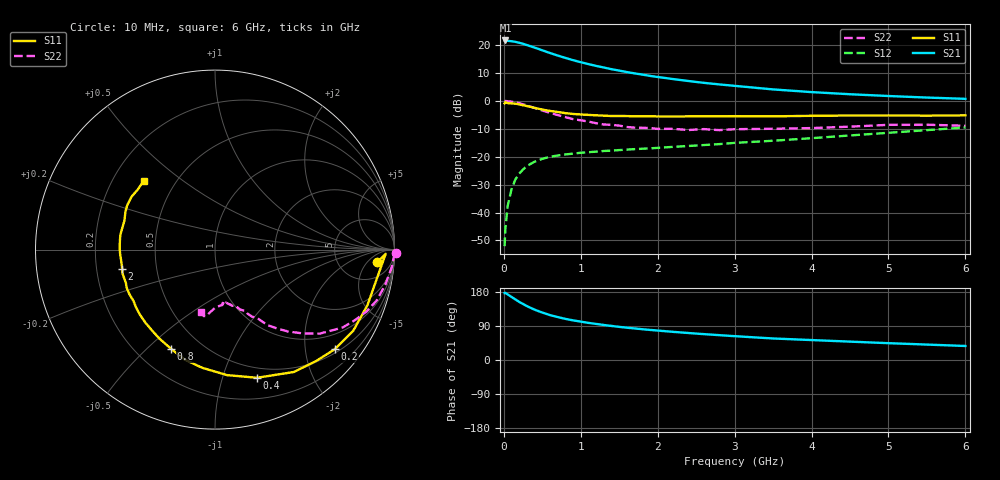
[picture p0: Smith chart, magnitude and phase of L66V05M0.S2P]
!  INFINEON TECHNOLOGIES Small Signal Semiconductors
! BFR380L3 , Si-NPN RF-Transistor in TSLP-3-1
!  Vce=6 V,  Ic=5 mA
! Common Emitter S-Parameters:  07. March 2005
#  GHz  S  MA  R  50
! f  S11  S21  S12  S22
! GHz  Mag  Ang  Mag  Ang  Mag  Ang  Mag  Ang
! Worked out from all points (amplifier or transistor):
!   36 points, 10 MHz to 6 GHz, reference 50 ohm
!   highest |S21| = 21.7 dB at 20 MHz (marker M1)
!   |S21| within 3 dB of that: start of sweep to 445.7 MHz
!   unconditionally stable (mu >= 1): 3.068 GHz to 4.502 GHz
!   at 250 MHz: K = 0.14, MSG = 22.5 dB, |S12| = -24.6 dB
!   at 1.4 GHz: K = 0.69, MSG = 14.6 dB, |S12| = -17.8 dB
!   at 6 GHz: K = 0.92, MSG = 5.1 dB, |S12| = -9.5 dB
!   S11 on the Smith chart (normalised r, x): 10 MHz: 13, -10; 200 MHz: 0.59, -2.65; 400 MHz: 0.40, -1.30; 800 MHz: 0.34, -0.60; 2 GHz: 0.31, -0.09; 6 GHz: 0.33, +0.37
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0.01  0.9068 -4.4  12.08 176.7  0.0025 71.3  1.011 -1.2
0.02  0.9514 -1.4  12.13 177.3  0.0051 91.3  0.997 -2.5
0.05  0.9152 -10.5  11.97 173.0  0.0132 85.6  0.9886 -6.0
0.1  0.9042 -20.0  11.73 166.4  0.0263 80.1  0.9685 -11.7
0.15  0.8932 -30.4  11.47 159.8  0.0393 73.9  0.9441 -17.5
0.2  0.8679 -39.8  11.04 153.3  0.0499 70.3  0.9115 -22.3
0.3  0.8112 -57.2  10.03 142.2  0.0683 61.6  0.8321 -31.5
0.4  0.7513 -71.9  9.044 132.8  0.0816 55.3  0.7475 -38.8
0.5  0.7025 -84.5  8.078 125.2  0.0919 51.1  0.674 -43.8
0.6  0.6626 -96.1  7.22 118.5  0.0999 47.4  0.6127 -48.2
0.7  0.6354 -105.5  6.509 113.3  0.1054 45.6  0.559 -51.8
0.8  0.6046 -113.8  5.908 108.5  0.11 43.4  0.5137 -55.1
0.9  0.5848 -121.9  5.379 104.6  0.1137 42.4  0.4729 -57.1
1.1  0.5623 -133.5  4.572 97.9  0.1207 41.6  0.4268 -61.1
1.5  0.538 -152.4  3.497 87.4  0.1317 42.1  0.3617 -67.3
2  0.5279 -168.4  2.688 77.7  0.1443 44.8  0.3158 -74.5
2.2  0.5265 -173.1  2.468 74.3  0.1505 45.9  0.3168 -74.9
2.8  0.5323 174.0  1.979 65.6  0.1685 50.4  0.3001 -81.9
3.5  0.5298 162.4  1.61 56.8  0.1937 53.6  0.3174 -87.5
4.5  0.5484 153.0  1.319 48.5  0.2408 58.5  0.3464 -93.9
5.5  0.5453 142.3  1.15 40.7  0.3001 59.8  0.3754 -99.7
6  0.552 135.8  1.091 37.0  0.3351 59.2  0.3584 -102.2
